(* Logix 5000 AddOnInstructionDefinition export ACS_SET_DIGITAL_OUTPUTS; software revision 20.01 *)

ADD_ON_INSTRUCTION ACS_SET_DIGITAL_OUTPUTS   (* revision 2.0, vendor Tolomatic, Inc *)
// Set Digital Output Bits on ACS Drive and Controller
VAR_IN_OUT
   DriveDigitalOutput : DINT; {required}   // ACS.0.DIGITAL_OUTPUT
END_VAR
VAR_INPUT
   DigitalOutput1 : BOOL; {visible}   // Digital Output 1
   DigitalOutput2 : BOOL; {visible}   // Digital Output 2
   DigitalOutput3 : BOOL; {visible}   // Digital Output 3
   DigitalOutput4 : BOOL; {visible}   // Digital Output 4
END_VAR
VAR
   DigitalOutputs : DINT; {access None}   // Combined value of the digital inputs
END_VAR

ROUTINE Logic   (* ladder *)
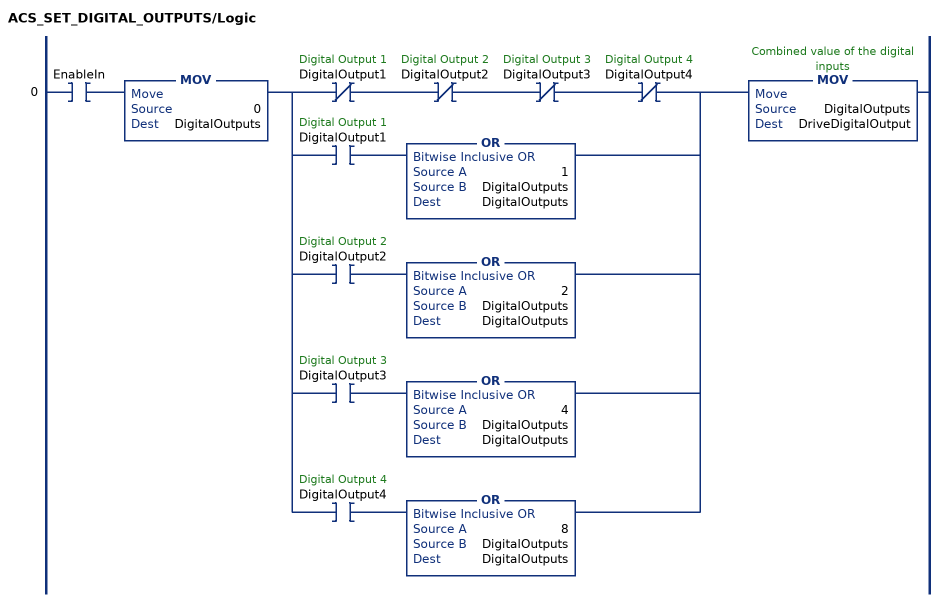
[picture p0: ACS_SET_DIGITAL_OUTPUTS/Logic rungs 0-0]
   0: XIC(EnableIn)MOV(0,DigitalOutputs)[XIO(DigitalOutput1) XIO(DigitalOutput2) XIO(DigitalOutput3) XIO(DigitalOutput4) ,XIC(DigitalOutput1) OR(1,DigitalOutputs,DigitalOutputs) ,XIC(DigitalOutput2) OR(2,DigitalOutputs,DigitalOutputs) ,XIC(DigitalOutput3) OR(4,DigitalOutputs,DigitalOutputs) ,XIC(DigitalOutput4) OR(8,DigitalOutputs,DigitalOutputs) ]MOV(DigitalOutputs,DriveDigitalOutput);
END_ROUTINE
END_ADD_ON_INSTRUCTION
